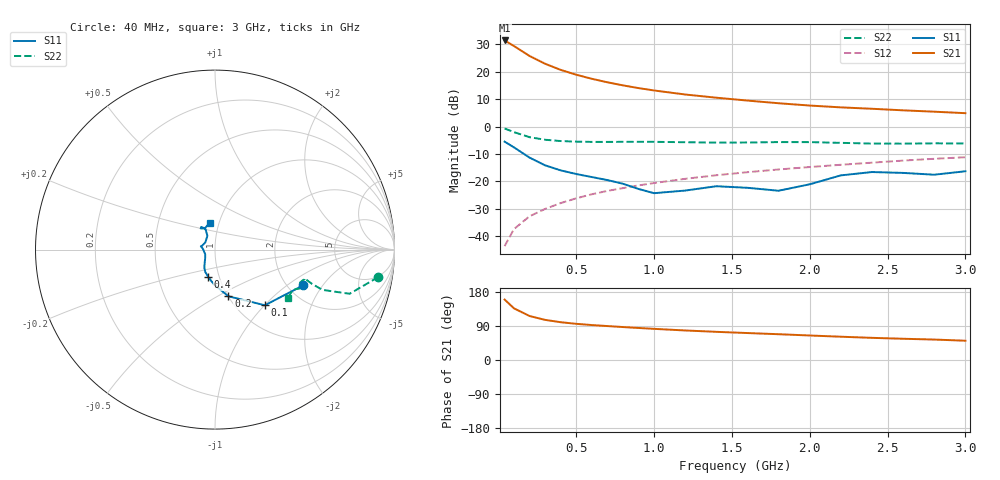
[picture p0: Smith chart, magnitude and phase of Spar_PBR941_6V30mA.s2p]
! Filename:  PBR941Q.S2P  Version:  3.0
! NXP part #:  PBR941  Date: July 1998
! Bias condition:  Vce=6V, Ic=30mA
#  MHz  S  MA  R 50
! Freq  S11  S21  S12  S22
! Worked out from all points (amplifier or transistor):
!   21 points, 40 MHz to 3 GHz, reference 50 ohm
!   highest |S21| = 31.4 dB at 40 MHz (marker M1)
!   |S21| within 3 dB of that: start of sweep to 126.7 MHz
!   unconditionally stable (mu >= 1): 548.8 MHz to 2.229 GHz
!   at 300 MHz: K = 0.91, MSG = 26.5 dB, |S12| = -30.1 dB
!   at 1 GHz: K = 1.04, MAG = 15.7 dB, |S12| = -20.6 dB
!   at 3 GHz: K = 0.97, MSG = 8.0 dB, |S12| = -11.2 dB
!   lowest NFmin = 2.69 dB at 500 MHz
!   S11 on the Smith chart (normalised r, x): 40 MHz: 2.40, -1.33; 100 MHz: 1.34, -1.00; 200 MHz: 1.00, -0.56; 400 MHz: 0.89, -0.28; 3 GHz: 0.91, +0.28
40  0.5292 -22.2  37.29 159.5  0.006528 80.2  0.9215 -9.6
100  0.4165 -48.1  29.52 136.4  0.01337 74.4  0.7893 -18.2
200  0.2706 -74.0  19.43 116.1  0.02295 73.7  0.639 -20.6
300  0.1955 -91.2  14 105.9  0.03124 76.3  0.5733 -19.5
400  0.1581 -103.7  10.83 99.7  0.03993 77.6  0.5429 -18.5
500  0.1357 -113.5  8.83 95.4  0.04881 78.8  0.529 -18.0
600  0.1194 -119.6  7.439 92.2  0.05788 79.5  0.5237 -17.8
700  0.1052 -123.9  6.423 89.5  0.06668 80.2  0.5235 -17.9
800  0.09018 -129.2  5.644 87.0  0.07499 80.6  0.525 -18.0
900  0.07241 -139.1  5.033 84.5  0.08408 80.5  0.5254 -18.2
1000  0.06058 -154.2  4.554 82.2  0.09286 80.4  0.5251 -18.4
1200  0.06767 176.2  3.844 77.9  0.1109 80.2  0.5166 -19.5
1400  0.08118 166.9  3.359 74.3  0.1289 79.7  0.5082 -21.2
1600  0.07599 164.2  2.977 71.1  0.1465 79.4  0.5108 -22.9
1800  0.0672 143.1  2.66 68.0  0.1643 79.1  0.5196 -24.1
2000  0.08808 118.6  2.415 64.7  0.182 78.3  0.5183 -24.8
2200  0.1282 114.8  2.237 61.4  0.2001 77.1  0.503 -25.8
2400  0.1475 121.3  2.11 58.5  0.2187 76.5  0.4883 -28.0
2600  0.1421 124.1  1.975 56.0  0.2386 75.9  0.4864 -30.9
2800  0.1318 115.6  1.865 53.9  0.2575 75.2  0.4931 -32.9
3000  0.1523 100.3  1.753 50.9  0.2749 74.0  0.4897 -33.5
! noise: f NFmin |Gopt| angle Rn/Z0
500  2.693  0.021  -140.4  0.278
900  2.762  0.124  -142.9  0.215
1000  2.831  0.098  -135.9  0.258
2000  3.554  0.269  -110.1  0.446
